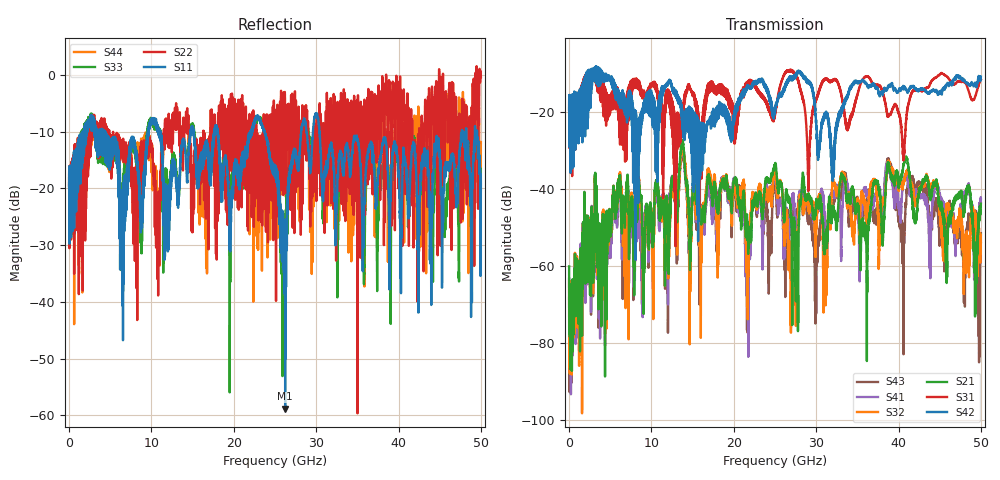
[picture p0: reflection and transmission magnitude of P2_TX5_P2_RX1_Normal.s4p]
!Keysight Technologies,N5225B,MY57041031,A.13.20.10
!Date: Friday, May 31, 2019 11:27:44
!Correction: S11(Full 4 Port(1,2,3,4))
!S12(Full 4 Port(1,2,3,4))
!S13(Full 4 Port(1,2,3,4))
!S14(Full 4 Port(1,2,3,4))
!S21(Full 4 Port(1,2,3,4))
!S22(Full 4 Port(1,2,3,4))
!S23(Full 4 Port(1,2,3,4))
!S24(Full 4 Port(1,2,3,4))
!S31(Full 4 Port(1,2,3,4))
!S32(Full 4 Port(1,2,3,4))
!S33(Full 4 Port(1,2,3,4))
!S34(Full 4 Port(1,2,3,4))
!S41(Full 4 Port(1,2,3,4))
!S42(Full 4 Port(1,2,3,4))
!S43(Full 4 Port(1,2,3,4))
!S44(Full 4 Port(1,2,3,4))
!S4P File: Measurements: <S11,S12,S13,S14>,
!<S21,S22,S23,S24>,
!<S31,S32,S33,S34>,
!<S41,S42,S43,S44>:
# Hz S  dB  R 50.0
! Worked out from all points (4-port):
!   5000 points, 10 MHz to 50 GHz, reference 50 ohm
!   strongest paths, dB at 10 MHz, 12.51 GHz, 25.01 GHz, 37.51 GHz, 50 GHz:
!     S42: -19.5, -14.1, -20.1, -14.3, -10.9
!     S31: -19.5, -17.8, -20.9, -13.1, -11.7
!     S21: -60.1, -37.6, -33.5, -38.4, -43.8
!     S32: -63.9, -38.5, -35.6, -48.4, -53.9
!     S41: -63.3, -37.5, -36.4, -40.5, -42.5
!     S43: -68.2, -38.2, -38.7, -44.7, -51.5
!   lowest |S11| = -58.8 dB at 26.24 GHz (marker M1), VSWR 1.00, Z = 49.9 + j0.0526 ohm
!   |S11| at or under -10 dB: 4.282 GHz to 9.568 GHz (5.286 GHz wide, 76.3 % of centre); 23.74 GHz to 28.18 GHz (4.439 GHz wide, 17.1 % of centre); 30.41 GHz to 47.7 GHz (17.29 GHz wide, 44.3 % of centre)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
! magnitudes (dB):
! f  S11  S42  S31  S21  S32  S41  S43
! 10 MHz  -19.8  -19.5  -19.5  -60.1  -63.9  -63.3  -68.2
! 13.77 GHz  -11.8  -20.0  -21.0  -27.4  -29.0  -28.6  -30.2
! 14.68 GHz  -10.6  -24.9  -13.8  -58.7  -62.6  -58.3  -56.2
! 26.24 GHz  -58.8  -13.6  -9.9  -43.9  -49.4  -48.6  -66.0
! 30 GHz  -6.9  -22.2  -16.7  -44.2  -50.2  -47.6  -72.4
! 38.77 GHz  -21.2  -13.3  -21.1  -33.3  -32.7  -34.0  -32.5
! 50 GHz  -19.3  -10.9  -11.7  -43.8  -53.9  -42.5  -51.5
